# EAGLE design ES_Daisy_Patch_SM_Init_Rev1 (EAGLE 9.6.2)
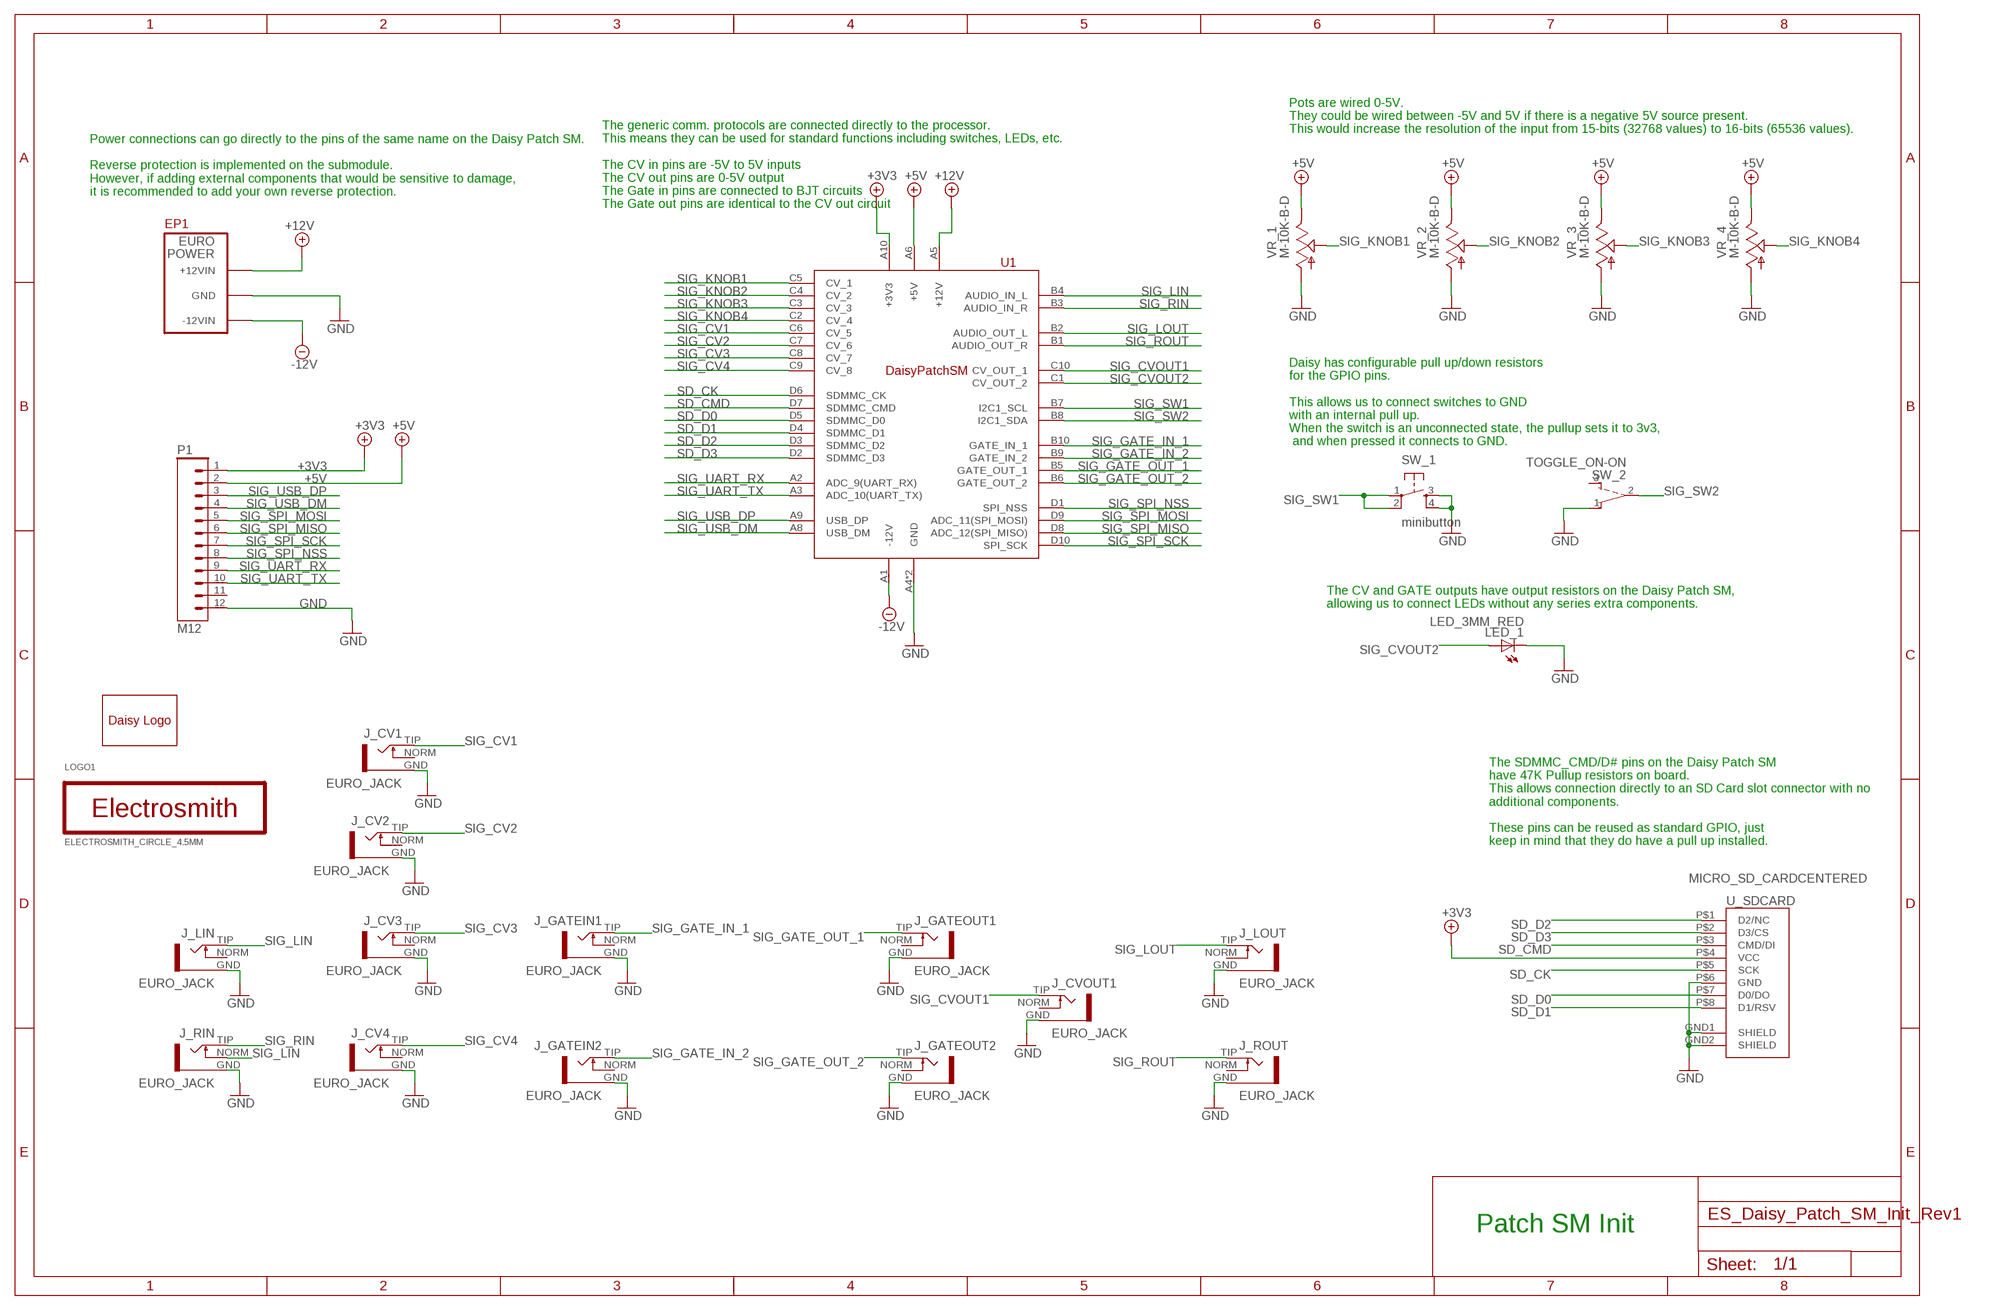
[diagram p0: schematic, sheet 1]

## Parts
EP1  EURORACK_POWERLOCK  [EURORACK_POWER_SHROUD_LOCK]
J_CV1  EURO_JACK  [S_JACK]
J_CV2  EURO_JACK  [S_JACK]
J_CV3  EURO_JACK  [S_JACK]
J_CV4  EURO_JACK  [S_JACK]
J_CVOUT1  EURO_JACK  [S_JACK]
J_GATEIN1  EURO_JACK  [S_JACK]
J_GATEIN2  EURO_JACK  [S_JACK]
J_GATEOUT1  EURO_JACK  [S_JACK]
J_GATEOUT2  EURO_JACK  [S_JACK]
J_LIN  EURO_JACK  [S_JACK]
J_LOUT  EURO_JACK  [S_JACK]
J_RIN  EURO_JACK  [S_JACK]
J_ROUT  EURO_JACK  [S_JACK]
LED_1  LED_3MM_RED  [LED]
LOGO1  ELECTROSMITH_CIRCLE_4.5MM  [ES_CIRCLE_4.5MM]
P1  M12  [1X12]
SW_1  minibutton  TAC_SWITCH_PTH_SILK  [TL1105SPF250Q_SILK]
SW_2  TOGGLE_ON-ON  [TOGGLE_ON-ON]
U1  ES_DAISY_PATCH_SM_REV1  [ES_DAISY_PATCH_SM_REV1]
U$2  DAISYLOGO  [ES_DAISY_LOGO_1]
U_SDCARD  MICRO_SD_CARDCENTERED  [VERT_MICROSD_CENTERED]
VR_1  M-10K-B-D  POT_9MM_SNAP-IN__  [9MM_SNAP-IN_POT_SILK]
VR_2  M-10K-B-D  POT_9MM_SNAP-IN__  [9MM_SNAP-IN_POT_SILK]
VR_3  M-10K-B-D  POT_9MM_SNAP-IN__  [9MM_SNAP-IN_POT_SILK]
VR_4  M-10K-B-D  POT_9MM_SNAP-IN__  [9MM_SNAP-IN_POT_SILK]

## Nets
+3V3 [power]: P1.1 U1.A10(+3V3) U_SDCARD.P$4(VCC)
+5V [power]: P1.2 U1.A6(+5V) VR_1.3 VR_2.3 VR_3.3 VR_4.3
+12V [power]: EP1.POS1(+12VIN) EP1.POS2(+12VIN) U1.A5(+12V)
-12V [power]: EP1.NEG1(-12VIN) EP1.NEG2(-12VIN) U1.A1(-12V)
GND [power]: EP1.GND1(GND) EP1.GND2(GND) EP1.GND3(GND) EP1.GND4(GND) EP1.GND5(GND) EP1.GND6(GND) J_CV1.GND J_CV2.GND J_CV3.GND J_CV4.GND J_CVOUT1.GND J_GATEIN1.GND J_GATEIN2.GND J_GATEOUT1.GND J_GATEOUT2.GND J_LIN.GND J_LOUT.GND J_RIN.GND J_ROUT.GND LED_1.K(C) P1.12 SW_1.3 SW_1.4 SW_2.1(O) U1.A4(GND) U1.A7(GND) U_SDCARD.GND1(SHIELD) U_SDCARD.GND2(SHIELD) U_SDCARD.P$6(GND) VR_1.1 VR_2.1 VR_3.1 VR_4.1
SD_CK: U1.D6(SDMMC_CK) U_SDCARD.P$5(SCK)
SD_CMD: U1.D7(SDMMC_CMD) U_SDCARD.P$3(CMD/DI)
SD_D0: U1.D5(SDMMC_D0) U_SDCARD.P$7(D0/DO)
SD_D1: U1.D4(SDMMC_D1) U_SDCARD.P$8(D1/RSV)
SD_D2: U1.D3(SDMMC_D2) U_SDCARD.P$1(D2/NC)
SD_D3: U1.D2(SDMMC_D3) U_SDCARD.P$2(D3/CS)
SIG_CV1: J_CV1.TIP U1.C6(CV_5)
SIG_CV2: J_CV2.TIP U1.C7(CV_6)
SIG_CV3: J_CV3.TIP U1.C8(CV_7)
SIG_CV4: J_CV4.TIP U1.C9(CV_8)
SIG_CVOUT1: J_CVOUT1.TIP U1.C10(CV_OUT_1)
SIG_CVOUT2: LED_1.A U1.C1(CV_OUT_2)
SIG_GATE_IN_1: J_GATEIN1.TIP U1.B10(GATE_IN_1)
SIG_GATE_IN_2: J_GATEIN2.TIP U1.B9(GATE_IN_2)
SIG_GATE_OUT_1: J_GATEOUT1.TIP U1.B5(GATE_OUT_1)
SIG_GATE_OUT_2: J_GATEOUT2.TIP U1.B6(GATE_OUT_2)
SIG_KNOB1: U1.C5(CV_1) VR_1.2
SIG_KNOB2: U1.C4(CV_2) VR_2.2
SIG_KNOB3: U1.C3(CV_3) VR_3.2
SIG_KNOB4: U1.C2(CV_4) VR_4.2
SIG_LIN: J_LIN.TIP J_RIN.NORM U1.B4(AUDIO_IN_L)
SIG_LOUT: J_LOUT.TIP U1.B2(AUDIO_OUT_L)
SIG_RIN: J_RIN.TIP U1.B3(AUDIO_IN_R)
SIG_ROUT: J_ROUT.TIP U1.B1(AUDIO_OUT_R)
SIG_SPI_MISO: P1.6 U1.D8(ADC_12(SPI_MISO))
SIG_SPI_MOSI: P1.5 U1.D9(ADC_11(SPI_MOSI))
SIG_SPI_NSS: P1.8 U1.D1(SPI_NSS)
SIG_SPI_SCK: P1.7 U1.D10(SPI_SCK)
SIG_SW1: SW_1.1 SW_1.2 U1.B7(I2C1_SCL)
SIG_SW2: SW_2.2(P) U1.B8(I2C1_SDA)
SIG_UART_RX: P1.9 U1.A2(ADC_9(UART_RX))
SIG_UART_TX: P1.10 U1.A3(ADC_10(UART_TX))
SIG_USB_DM: P1.4 U1.A8(USB_DM)
SIG_USB_DP: P1.3 U1.A9(USB_DP)
Unconnected: J_CV1.NORM J_CV2.NORM J_CV3.NORM J_CV4.NORM J_CVOUT1.NORM J_GATEIN1.NORM J_GATEIN2.NORM J_GATEOUT1.NORM J_GATEOUT2.NORM J_LIN.NORM J_LOUT.NORM J_ROUT.NORM P1.11 SW_2.3(S)

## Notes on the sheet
- Pots are wired 0-5V.
  They could be wired between -5V and 5V if there is a negative 5V source present. 
  This would increase the resolution of the input from 15-bits (32768 values) to 16-bits (65536 values).
- Power connections can go directly to the pins of the same name on the Daisy Patch SM.
  
  Reverse protection is implemented on the submodule. 
  However, if adding external components that would be sensitive to damage, 
  it is recommended to add your own reverse protection.
- The generic comm. protocols are connected directly to the processor.
  This means they can be used for standard functions including switches, LEDs, etc.
  
  The CV in pins are -5V to 5V inputs
  The CV out pins are 0-5V output
  The Gate in pins are connected to BJT circuits
  The Gate out pins are identical to the CV out circuit
- EP1
- Daisy has configurable pull up/down resistors 
  for the GPIO pins.
  
  This allows us to connect switches to GND
  with an internal pull up. 
  When the switch is an unconnected state, the pullup sets it to 3v3,
   and when pressed it connects to GND.
- The CV and GATE outputs have output resistors on the Daisy Patch SM,
  allowing us to connect LEDs without any series extra components.
- The SDMMC_CMD/D# pins on the Daisy Patch SM 
  have 47K Pullup resistors on board.
  This allows connection directly to an SD Card slot connector with no 
  additional components.
  
  These pins can be reused as standard GPIO, just 
  keep in mind that they do have a pull up installed.
- Patch SM Init

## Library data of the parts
EP1 = Electrosmith-Connectors:EURORACK_POWER; MPN: 2x5x.1-header
J_CV1-J_CV4 J_CVOUT1 J_GATEIN1 J_GATEIN2 J_GATEOUT1 J_GATEOUT2 J_LIN J_LOUT J_RIN J_ROUT = Electrosmith-Interface:EURO_JACK
LED_1 = Electrosmith-Interface:LED; COLOR: RED; SIZE: 3MM
LOGO1 = Electrosmith-Logo:ELECTROSMITH
P1 = Electrosmith-Connectors:M12
SW_1 = Electrosmith-Interface:TAC_SWITCH_PTH: Momentary Switch Button commonly used for reset or general input. Spark Fun Electronics SKU : COM-00097; IPN: Mini Button; MPN: TL1105SPF250Q
SW_2 = Electrosmith-Interface:TOGGLE_ON-ON
U1 = Electrosmith-Boards:ES_DAISY_PATCH_SM_REV1
U$2 = Electrosmith-Logo:DAISYLOGO
U_SDCARD = Electrosmith-Interface:MICRO_SD_CARD
VR_1-VR_4 = Electrosmith-Interface:POT_9MM_SNAP-IN_: 9mm vertical snap-in pot, Alpha / Panasonic style

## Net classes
0 default: width 0.203 mm, clearance 0.254 mm
1 power: width 0.406 mm, clearance 0.406 mm

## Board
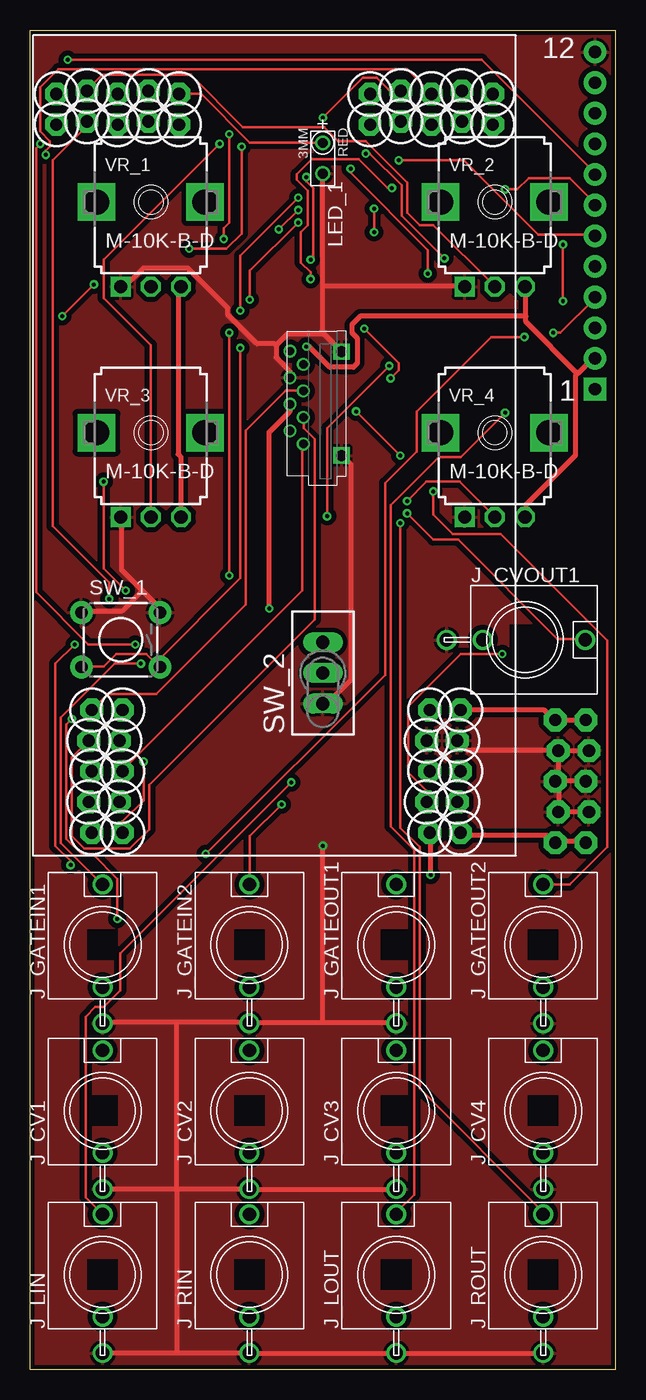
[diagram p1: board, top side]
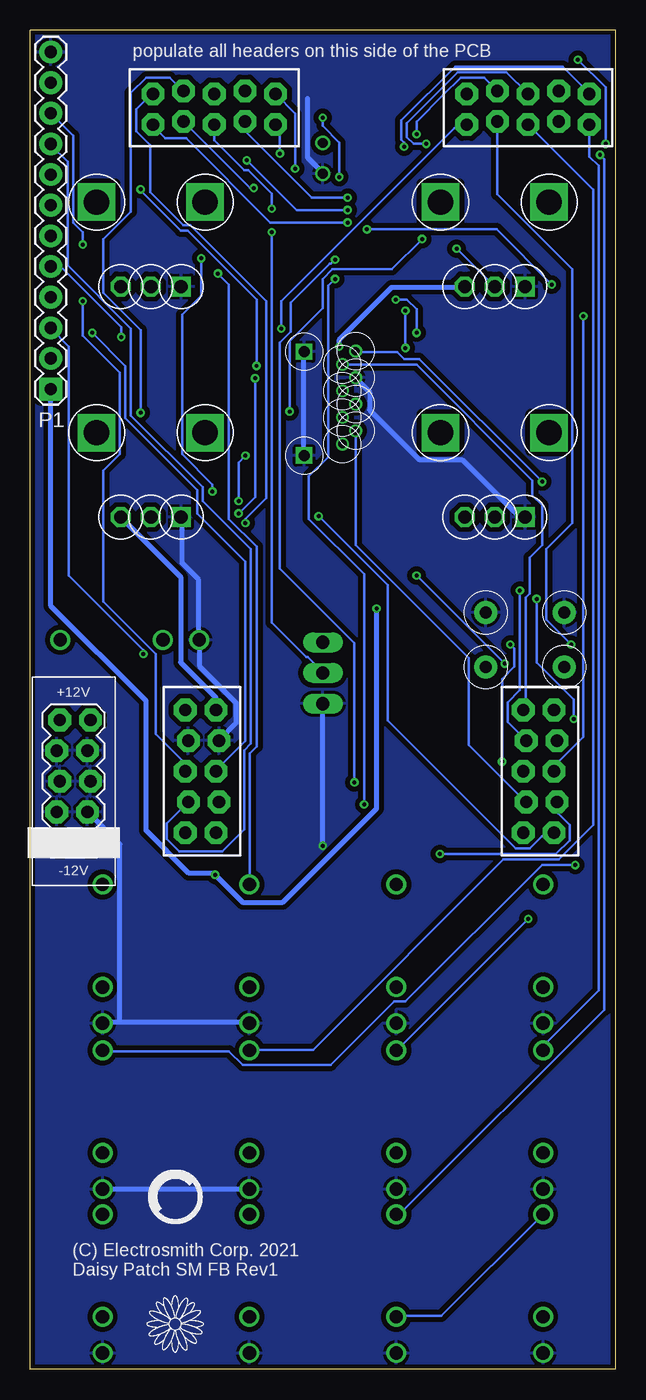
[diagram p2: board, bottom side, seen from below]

Size 48.5 x 111 mm. Coordinates in mm from the lower left corner, seen from the top.
Outline: 0,0 48.5,0 48.5,111 0,111 0,0
Copper layers (1*16): Top 0.0356mm / dielectric 1.5011mm / Bottom 0.0356mm
Design rules "ES_DRC_MaskedVias": minimum track width 6mil, minimum drill 13mil, track to track 6mil, track to pad 6mil, pad to pad 6mil, via to via 6mil, smd to smd 6mil, copper to edge 15mil, drill to drill 6mil, minimum pad ring 7mil, minimum via ring 7mil, stop-mask expansion 3mil, vias tented up to drill 16mil, thermal gap 10mil

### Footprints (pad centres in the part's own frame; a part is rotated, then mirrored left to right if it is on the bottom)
EURORACK_POWER_SHROUD_LOCK = drill 1.016 pad 1.88 octagon: GND1 -2.54,1.143; GND2 -2.54,-1.397; GND3 0,1.397; GND4 0,-1.143; GND5 2.54,1.143; GND6 2.54,-1.397; NEG1 5.08,1.397; NEG2 5.08,-1.143; POS1 -5.08,1.397; POS2 -5.08,-1.143
S_JACK = drill 1.1: GND 0,-6.5; NORM 0,-3.5; TIP 0,5
LED = drill 0.813: A -1.27,0; K 1.27,0
1X12 = drill 1.016 pad 1.88 square: 1 0,0 | drill 1.016 pad 1.88: 2 2.54,0; 3 5.08,0; 4 7.62,0; 5 10.16,0; 6 12.7,0; 7 15.24,0; 8 17.78,0; 9 20.32,0; 10 22.86,0; 11 25.4,0; 12 27.94,0
TL1105SPF250Q_SILK = drill 1.016 pad 1.88: 1 -3.251,2.261; 2 3.251,2.261; 3 -3.251,-2.261; 4 3.251,-2.261
TOGGLE_ON-ON = drill 1.1 pad 1.422 long: 1 -2.54,0; 2 0,0; 3 2.54,0
ES_DAISY_PATCH_SM_REV1 = drill 1.016 pad 1.88 octagon: A1 -32.08,-15.397; A2 -29.54,-15.143; A3 -27,-15.397; A4 -24.46,-15.143; A5 -21.92,-15.397; A6 -21.92,-12.857; A7 -24.46,-12.603; A8 -27,-12.857; A9 -29.54,-12.603; A10 -32.08,-12.857; B1 29.143,-18.08; B2 29.397,-15.54; B3 29.143,-13; B4 29.397,-10.46; B5 29.143,-7.92; B6 26.603,-7.92; B7 26.857,-10.46; B8 26.603,-13; B9 26.857,-15.54; B10 26.603,-18.08; C1 29.143,7.92; C2 29.397,10.46; C3 29.143,13; C4 29.397,15.54; C5 29.143,18.08; C6 26.603,18.08; C7 26.857,15.54; C8 26.603,13; C9 26.857,10.46; C10 26.603,7.92; D1 -32.08,12.603; D2 -29.54,12.857; D3 -27,12.603; D4 -24.46,12.857; D5 -21.92,12.603; D6 -21.92,15.143; D7 -24.46,15.397; D8 -27,15.143; D9 -29.54,15.397; D10 -32.08,15.143
VERT_MICROSD_CENTERED = drill 0.9 square: GND1 -3.9,-1.55; GND2 4.7,-1.55 | drill 0.7: P$1 -2.95,1.62; P$2 -1.85,2.72; P$3 -0.75,1.62; P$4 0.35,2.72; P$5 1.45,1.62; P$6 2.55,2.72; P$7 3.65,1.62; P$8 4.75,2.72
9MM_SNAP-IN_POT_SILK = drill 1.1 square: 1 -2.5,-7 | drill 1.1 octagon: 2 0,-7; 3 2.5,-7 | drill 2.1 square: CHASSIS1 -4.5,0; CHASSIS2 4.5,0

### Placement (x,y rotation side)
EP1  44.9,48.74 270 bottom
J_CV1  6,21.44 0 top
J_CV2  18.17,21.44 0 top
J_CV3  30.33,21.44 0 top
J_CV4  42.5,21.44 0 top
J_CVOUT1  41,60.47 270 top
J_GATEIN1  6,35.19 0 top
J_GATEIN2  18.17,35.19 0 top
J_GATEOUT1  30.33,35.19 0 top
J_GATEOUT2  42.5,35.19 0 top
J_LIN  6,7.85 0 top
J_LOUT  30.33,7.85 0 top
J_RIN  18.17,7.85 0 top
J_ROUT  42.5,7.85 0 top
LED_1  24.25,100.38 270 top
LOGO1  36.5,14.25 0 bottom
P1  46.8,81.25 90 bottom
SW_1  7.5,60.47 180 top
SW_2  24.25,57.72 90 top
U1  20.25,76.57 90 top
U$2  36.5,3.75 0 bottom
U_SDCARD  24.25,79.65 90 top
VR_1  10,96.75 0 top
VR_2  38.5,96.75 0 top
VR_3  10,77.64 0 top
VR_4  38.5,77.64 0 top

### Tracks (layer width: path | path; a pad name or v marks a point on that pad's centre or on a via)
+3V3  (via drill 0.33)
  Top 0.406: v19.8,63.06 19.8,77.69 21.52,79.4 21.52,79.97 U_SDCARD.P$4 | U1.A10 33.18,44.42 v33.18,41
  Bottom 0.406: v19.8,63.06 19.8,46.48 27.57,38.71 30.89,38.71 v33.18,41 33.29,41.11 35.35,41.11 38.89,44.66 38.89,55.4 46.78,63.29 46.78,81.23 P1.1
+5V  (via drill 0.33)
  Top 0.406: VR_3.3 12.49,70.72 12.49,75.63 12.26,75.86 12.26,89.46 12.49,89.69 VR_1.3 | 45.35,82.55 45.18,82.37 45.18,75.75 41.06,71.63 41.06,70.72 VR_4.3 | 41.06,87.29 41.06,86.83 45.35,82.55 | 41.06,87.29 41.06,89.69 VR_2.3 | v22.89,84.77 23.12,84.77 24.83,83.06 26.77,83.06 27.12,83.4 27.12,85.46 26.66,85.92 26.66,86.6 27.35,87.29 41.06,87.29 | P1.2 46.6,83.79 45.35,82.55
  Bottom 0.406: VR_4.3 40.95,70.6 36.03,65.69 36.03,58.6 33.11,55.67 U1.A6 | v22.89,84.77 22.89,85.35 18.55,89.69 12.6,89.69 VR_1.3
+12V
  Top 0.406: EP1.POS2 45.98,53.8 43.58,53.8 EP1.POS1 43.35,53.91 42.61,54.65 U1.A5
-12V
  Top 0.406: EP1.NEG2 45.98,43.74 43.58,43.74 EP1.NEG1 43.35,43.74 42.82,44.27 35.87,44.27 U1.A1
GND  (via drill 0.33)
  Top 0.406: 9.29,64.54 10.66,63.17 10.66,62.83 SW_1.3 | 9.29,64.54 7.57,66.26 7.57,70.6 VR_3.1 | 9.29,64.54 7.57,62.83 4.26,62.83 SW_1.4 | 20.37,84.89 20.37,83.86 21.52,82.72 21.52,82.26 U_SDCARD.P$6 | 20.37,84.89 21.29,85.8 24.26,85.8 | 24.26,85.8 24.38,85.8 25.75,84.43 U_SDCARD.GND2 | 24.26,85.8 24.26,89.8 | 24.26,89.8 24.26,99.06 LED_1.K | SW_2.1 24.26,55.28 24.72,55.28 26.55,57.11 26.55,75.06 25.86,75.75 U_SDCARD.GND1 | VR_1.1 7.57,89.8 7.91,89.8 9.4,91.29 13.06,91.29 16.37,87.97 16.37,87.4 18.77,85 20.26,85 20.37,84.89 | 24.26,89.8 35.92,89.8 VR_2.1 | EP1.GND3 43.58,48.77 45.98,48.77 EP1.GND4 | EP1.GND3 43.81,48.66 43.81,46.25 EP1.GND5 43.92,46.25 46.21,46.25 EP1.GND6 | EP1.GND1 43.81,51.17 43.81,48.88 EP1.GND3 | EP1.GND2 46.21,51.28 43.92,51.28 EP1.GND1 | EP1.GND1 43.58,51.28 36.22,51.28 U1.A4 | 12.14,28.77 18.09,28.77 J_GATEIN2.GND 18.32,28.77 24.26,28.77 | 12.14,28.77 6.09,28.77 J_GATEIN1.GND | 24.26,28.77 30.32,28.77 J_GATEOUT1.GND | 12.14,1.33 18.09,1.33 J_RIN.GND 18.32,1.33 30.32,1.33 J_LOUT.GND 30.43,1.33 42.43,1.33 J_ROUT.GND | 12.14,1.33 6.09,1.33 J_LIN.GND | 12.14,14.94 18.09,14.94 J_CV2.GND 18.32,14.94 30.32,14.94 J_CV3.GND | 12.14,14.94 6.09,14.94 J_CV1.GND | 12.14,14.94 12.14,1.33 | 12.14,14.94 12.14,28.77 | 24.26,28.77 v24.26,43.4
  Bottom 0.406: U_SDCARD.GND1 25.86,75.86 25.86,84.32 U_SDCARD.GND2 | 25.52,105.35 25.52,100.43 24.26,99.18 LED_1.K | VR_3.1 7.57,70.72 8.03,70.72 12.72,75.4 16.26,75.4 20.37,79.52 20.37,81 21.52,82.15 U_SDCARD.P$6 | VR_4.1 35.92,70.6 35.92,66.83 34.55,65.46 34.55,60.66 J_CVOUT1.GND 34.43,60.43 34.43,58.26 31.46,55.28 31.46,53.57 32.85,52.18 U1.A7 | 41.06,28.77 30.43,28.77 J_GATEOUT1.GND | 41.06,28.77 42.43,28.77 J_GATEOUT2.GND | J_CV4.GND 42.43,14.94 30.43,14.94 J_CV3.GND | 41.06,28.77 41.06,43.51 43.69,46.14 EP1.GND5 | v24.26,43.4 SW_2.1
  pour Top: 0.2,110.85 0.2,0.25 48.3,0.25 48.3,110.55 48.3,110.85
  pour Bottom: 0.5,110.75 0.5,0.25 48,0.25 48,110.25 48,110.75
SD_CK
  Top 0.203: U_SDCARD.P$5 22.55,81.12 21.17,81.12 17.86,77.8 17.86,63.4 10.43,55.97 6.43,55.97 U1.D6
SD_CMD
  Top 0.203: U_SDCARD.P$3 22.66,78.83 22.66,78.03 23.57,77.12 23.57,62.14 9.86,48.43 9.86,44.77 8.26,43.17 4.49,43.17 3.46,44.2 3.46,50.72 U1.D7
SD_D0
  Bottom 0.203: U_SDCARD.P$7 22.55,83.29 16.49,83.29 6.89,73.69 6.89,72.43 6.09,71.63 6.09,68.31 7.12,67.29 7.12,64.31 7.46,63.97 7.46,54.84 U1.D5
SD_D1  (via drill 0.33)
  Top 0.203: v6.09,73.57 6.09,66.37 v7.91,64.54
  Bottom 0.203: v6.09,73.57 16.26,83.75 17.52,83.75 18.09,84.32 21.52,84.32 U_SDCARD.P$8 | v7.91,64.54 7.91,56.31 8.94,55.28 8.94,53.71 8.94,53.69 8.94,53.66 U1.D4
SD_D2
  Top 0.203: U_SDCARD.P$1 22.55,76.66 22.55,64.54 7.65,49.64 U1.D3
SD_D3
  Bottom 0.203: U_SDCARD.P$2 21.52,77.69 21.52,68.31 12.14,58.94 12.14,51.74 7.43,47.03 U1.D2
SIG_CV1
  Bottom 0.203: J_CV1.TIP 5.97,26.48 5.97,26.82 1.4,31.4 1.4,99.75 2.17,100.52 U1.C6
SIG_CV2  (via drill 0.33)
  Top 0.203: v7.23,37.34 7.23,40.65 5.17,42.71 4.26,42.71 3,43.97 3,53.46 v3.46,53.91 | v6.54,63.86 6.54,65.23 1.86,69.91 1.86,100.2 4.6,102.95 4.6,103.32 U1.C7
  Bottom 0.203: v7.23,37.34 18.09,26.48 J_CV2.TIP | v3.46,53.91 3.46,55.51 6.54,58.6 v6.54,63.86
SIG_CV3
  Bottom 0.203: J_CV3.TIP 30.32,26.48 25.06,26.48 9.29,42.25 4.71,42.25 1.86,45.11 1.86,97.78 U1.C8
SIG_CV4  (via drill 0.33)
  Top 0.203: v3.34,41.8 3.34,42.14 2.09,43.4 2.09,58.48 v3.69,60.09
  Bottom 0.203: v3.34,41.8 6.09,41.8 17.4,30.48 18.32,30.48 23.57,25.22 30.89,25.22 32.03,26.37 42.43,26.37 J_CV4.TIP | v3.69,60.09 5.74,62.14 5.74,67.97 3.57,70.14 3.57,91.17 9.79,97.39 U1.C9
SIG_CVOUT1  (via drill 0.33)
  Top 0.203: v31.23,70.94 33.4,68.77 35.46,68.77 43.69,60.54 45.98,60.54 J_CVOUT1.TIP | v29.86,82.15 30.55,82.83 30.55,83.4 v27.69,86.26
  Bottom 0.203: v31.23,70.94 29.86,72.32 v29.86,82.15 | v27.69,86.26 27.69,88.55 13.38,102.86 13.17,103.06 13.06,103.17 U1.C10
SIG_CVOUT2
  Top 0.203: LED_1.A 24.15,101.69 18.2,101.69 14.18,105.71 U1.C1
SIG_GATE_IN_1  (via drill 0.33)
  Top 0.203: v9.17,58.48 7,58.48 2.54,54.03 2.54,43.63 5.97,40.2 J_GATEIN1.TIP | v16.49,85.92 v16.49,65.8 | v18.2,88.66 18.2,91.06 v22.2,95.06
  Bottom 0.203: v16.49,65.8 v9.17,58.48 | v16.49,85.92 16.49,87.86 17.29,88.66 v18.2,88.66 | v22.2,95.06 28.6,95.06 35.58,102.03 37.29,102.03 38.33,103.07 U1.B10
SIG_GATE_IN_2  (via drill 0.33)
  Top 0.203: v20.83,46.83 18.2,44.2 18.2,40.2 J_GATEIN2.TIP | v23.23,90.38 23.23,90.95 22.43,91.75 22.43,94.26 23,94.83 23,97.69 22.09,98.61 22.09,99.06 23.35,100.32 27.23,100.32 29.63,97.92 v29.98,97.92
  Bottom 0.203: v20.83,46.83 20.83,65.91 25.4,70.49 25.4,74.03 23.8,75.63 23.8,89.8 v23.23,90.38 | U1.B9 30.28,97.92 v29.98,97.92
SIG_GATE_OUT_1  (via drill 0.33)
  Top 0.203: v32.95,90.83 32.95,92.78 26.55,99.18 v26.55,99.52
  Bottom 0.203: v32.95,90.83 32.03,89.92 32.03,70.49 29.75,68.2 29.75,51.63 30.32,51.06 30.32,40.2 J_GATEOUT1.TIP | v26.55,99.52 26.55,104.09 U1.B5
SIG_GATE_OUT_2  (via drill 0.33)
  Top 0.203: v33.4,72.77 33.4,70.83 35.01,69.23 39.01,69.23 47.81,60.43 47.81,43.28 44.72,40.2 42.55,40.2 J_GATEOUT2.TIP | v34.32,92.09 30.77,95.63 30.77,98.15 28.15,100.78 v27.8,100.78
  Bottom 0.203: v33.4,72.77 33.4,73.34 35.92,75.86 35.92,87.4 34.32,89 v34.32,92.09 | v27.8,100.78 27.8,102.72 28.17,103.09 U1.B6
SIG_KNOB1  (via drill 0.33)
  Top 0.203: v13.17,92.89 16.26,92.89 17.52,94.15 v17.52,101.35
  Bottom 0.203: v13.17,92.89 10.09,89.8 VR_1.2 | v17.52,101.35 17.52,101.69 17.75,101.92 17.75,103.52 13.29,107.98 4.37,107.98 2.17,105.78 U1.C5
SIG_KNOB2
  Top 0.203: VR_2.2 38.43,89.8 33.4,94.83 32.26,94.83 31.23,95.86 31.23,98.38 27.8,101.81 25.52,101.81 24.38,102.95 17.63,102.95 13.29,107.29 5.97,107.29 4.71,106.03 U1.C4
SIG_KNOB3  (via drill 0.33)
  Top 0.203: v15.69,101.58 6.09,91.97 6.09,88.78 9.97,84.89 9.97,70.72 VR_3.2
  Bottom 0.203: v15.69,101.58 16.72,101.58 17.29,102.15 17.29,103.29 13.06,107.52 9.06,107.52 U1.C3
SIG_KNOB4  (via drill 0.33)
  Top 0.203: v31.23,71.97 32.83,73.57 35.58,73.57 38.43,70.72 VR_4.2 | v27,79.4 v30.66,75.75 | v16.03,93.69 16.03,94.6 16.49,95.06 v16.49,102.38
  Bottom 0.203: v31.23,71.97 31.23,75.17 v30.66,75.75 | v27,79.4 27,85.23 24.26,87.97 24.26,90.38 23.46,91.17 18.55,91.17 v16.03,93.69 | v16.49,102.38 16.49,103.41 14.26,105.64 12.83,107.06 10.89,107.06 U1.C2
SIG_LIN  (via drill 0.33)
  Top 0.203: v24.26,103.75 27.57,107.06 28.72,107.06 29.66,106.12 29.75,106.03 29.81,105.97 U1.B4 | v22.89,98.83 22.89,98.49 23.46,97.92 23.46,92.2 v23.23,91.97 | v21.63,48.66 7.46,34.48 7.46,31.4 6.09,30.03 5.4,30.03 4.6,29.22 4.6,14.25 5.97,12.88 J_LIN.TIP
  Bottom 0.203: J_RIN.NORM 18.09,4.42 14.43,4.42 6.09,12.77 J_LIN.TIP | v24.26,103.75 24.26,103.06 22.89,101.69 v22.89,98.83 | v23.23,91.97 23.57,91.63 23.69,91.63 26.89,88.43 26.89,86.03 27.8,85.12 27.8,66.37 21.63,60.2 v21.63,48.66
SIG_LOUT  (via drill 0.33)
  Top 0.203: v39.35,79.29 35.69,75.63 33.86,75.63 29.86,71.63 29.86,45 31.8,43.06 31.8,14.48 30.43,13.11 30.43,12.88 J_LOUT.TIP
  Bottom 0.203: v39.35,79.29 39.35,86.15 42.43,89.23 42.43,93.69 40.15,95.98 40.15,105.81 38.89,107.06 36.94,107.06 35.85,105.97 U1.B2
SIG_RIN  (via drill 0.33)
  Top 0.203: v1.29,100.66 1.29,101 1.63,101.35 1.63,101.81 0.83,102.61 0.83,106.26 2.31,107.75 31.23,107.75 33.25,105.73 U1.B3
  Bottom 0.203: v1.29,100.66 0.94,100.32 0.94,29.8 17.86,12.88 18.09,12.88 J_RIN.TIP
SIG_ROUT  (via drill 0.33)
  Top 0.203: v30.66,70.14 30.66,44.88 32.26,43.28 32.26,23.28 42.43,13.11 42.43,12.88 J_ROUT.TIP
  Bottom 0.203: v30.66,70.14 30.66,70.49 28.95,72.2 28.95,88.55 35.23,94.83 35.8,94.83 38.55,97.58 38.55,101.46 39.69,102.61 39.69,104.43 38.41,105.71 U1.B1
SIG_SPI_MISO  (via drill 0.33)
  Top 0.203: v5.29,89.92 v2.66,87.29 | v22.2,96.09 v20.6,94.49 | v30.55,100.2 35.92,100.2 42.09,94.03 46.72,94.03 P1.6
  Bottom 0.203: v2.66,87.29 2.66,52.43 5.11,49.98 U1.D8 | v5.29,89.92 9.86,94.49 v20.6,94.49 | v22.2,96.09 26.43,96.09 v30.55,100.2
SIG_SPI_MOSI  (via drill 0.33)
  Top 0.203: v14.54,42.71 29.4,57.57 29.4,73.46 32.03,76.09 32.03,79.4 38.2,85.57 v40.95,85.57
  Bottom 0.203: v14.54,42.71 4.94,42.71 3.8,43.86 3.8,45.11 4.75,46.06 4.75,46.92 U1.D9 | v40.95,85.57 40.95,86.37 45.98,91.4 P1.5
SIG_SPI_NSS  (via drill 0.33)
  Top 0.203: v9.4,50.37 9.4,47.17 7.65,45.42 U1.D1 | v8.72,60.09 4.83,60.09 0.49,64.43 0.49,101.23 v0.83,101.58 | v3.12,108.55 37.41,108.55 46.8,99.15 P1.8
  Bottom 0.203: v9.4,50.37 9.4,57.23 8.37,58.26 8.37,59.74 v8.72,60.09 | v0.83,101.58 0.83,106.26 v3.12,108.55
SIG_SPI_SCK  (via drill 0.33)
  Top 0.203: v24.6,70.72 24.6,78.03 v29.75,83.17 | v39.35,97.8 40.38,97.8 41.29,98.72 44.72,98.72 46.26,97.18 46.26,97.03 P1.7
  Bottom 0.203: v24.6,70.72 18.89,65 18.89,53.8 8.26,43.17 7.12,43.17 6.12,44.16 5.86,44.43 5.79,44.49 U1.D10 | v29.75,83.17 29.75,88.66 35.46,94.38 36.03,94.38 39.35,97.69 v39.35,97.8
SIG_SW1  (via drill 0.33)
  Top 0.203: SW_1.2 4.26,58.26 6.09,58.26 7.12,59.28 9.63,59.28 10.66,58.26 SW_1.1 10.43,58.6 17.4,65.57 v17.4,84.66 | v22.2,97.12 17.4,92.32 v17.4,87.75
  Bottom 0.203: v22.2,97.12 25.18,97.12 30.71,102.65 U1.B7 | v17.4,84.66 v17.4,87.75
SIG_SW2  (via drill 0.33)
  Top 0.203: v28.49,96.2 v28.49,94.26
  Bottom 0.203: v28.49,94.26 28.49,61.91 25.63,59.06 25.52,59.06 24.26,57.8 SW_2.2 | v28.49,96.2 28.49,97.46 30.43,99.41 30.77,99.41 33.25,101.88 U1.B8
SIG_UART_RX
  Bottom 0.203: P1.9 46.8,101.48 45.41,100.09 45.41,91.52 40.15,86.26 40.15,79.06 34.2,73.12 34.2,71.97 30.2,67.97 30.2,51.86 30.77,51.28 30.77,44.77 32.6,42.94 36.15,42.94 37.18,43.97 37.18,45.25 U1.A2
SIG_UART_TX  (via drill 0.33)
  Top 0.203: v44.15,93.23 v44.15,88.55
  Bottom 0.203: v44.15,88.55 44.15,85.69 41.06,82.6 41.06,75.86 42.43,74.49 42.43,63.63 38.09,59.28 38.09,52.66 35.65,50.21 U1.A3 | v44.15,93.23 44.15,94.26 44.95,95.06 44.95,102.26 P1.10
SIG_USB_DM  (via drill 0.33)
  Top 0.203: v43.35,85.92 43.92,85.92 46.8,88.8 P1.4
  Bottom 0.203: v43.35,85.92 40.6,83.17 40.6,78.83 34.66,72.89 34.66,70.94 30.66,66.94 30.66,52.08 33.11,49.64 U1.A8
SIG_USB_DP  (via drill 0.33)
  Top 0.203: v39.12,59.28 35.69,59.28 31.35,54.94 31.35,49.46 32.85,47.95 U1.A9
  Bottom 0.203: v39.12,59.28 39.12,59.63 45.29,65.8 45.29,84.77 46.8,86.28 P1.3

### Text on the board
tPlace: 12 | 1
bPlace: populate all headers on this side of the PCB | (C) Electrosmith Corp. 2021 / Daisy Patch SM FB Rev1
_tNames: VR_1 | VR_2 | LED_1 | VR_3 | VR_4 | P1 | SW_1 | J_CVOUT1 | SW_2 | J_GATEIN1 | J_GATEIN2 | J_GATEOUT1 | J_GATEOUT2 | J_CV1 | J_CV2 | J_CV3 | J_CV4 | J_LIN | J_RIN | J_LOUT | J_ROUT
